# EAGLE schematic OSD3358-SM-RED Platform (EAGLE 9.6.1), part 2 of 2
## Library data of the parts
C1-C10 C12-C68 C70-C101 = OSD3358-SM-RED Platform:C: Capacitor SMD.
C11 C69 = OSD3358-SM-RED Platform:CPOL-US: POLARIZED CAPACITOR, American symbol
D1 D4-D7 D10 = OSD3358-SM-RED Platform:LTST-C191TBKT
D2 = OSD3358-SM-RED Platform:SMCJ15CA
D3 = OSD3358-SM-RED Platform:B520C-13-F: Schottky barrier diode
D8 D9 = OSD3358-SM-RED Platform:TPD4E05U06-Q1
D11 = OSD3358-SM-RED Platform:RB751V40-115
F1 = OSD3358-SM-RED Platform:FUSE
FB1 FB2 FB4 FB5 = OSD3358-SM-RED Platform:BLM21AG151SN1D: INDUCTOR
FB3 FB6 = OSD3358-SM-RED Platform:MPZ2012S601AT000: INDUCTOR
FUD1-FUD6 = OSD3358-SM-RED Platform:FIDUCIAL
J1 J2 J7-J9 J11 J12 J15 = OSD3358-SM-RED Platform:826646-2: 2-pin 100 mil header
J3 = OSD3358-SM-RED Platform:826646-6: 6-pin 100 mil header; MPN: P125-1106A1BS116A1
J4 = OSD3358-SM-RED Platform:FTR-110-51-L-D-06
J5 J6 = OSD3358-SM-RED Platform:TH-2X23: 320030002
J10 = OSD3358-SM-RED Platform:TH-2X5: 320030002
J14 = OSD3358-SM-RED Platform:PJ-102BH: 2.5 mm Center Pin, 5.0 A, Right Angle, Through Hole, Tapered Pins, Dc Power Jack Connector
L1 = OSD3358-SM-RED Platform:CVH252009-4R7M
MGT1-MGT4 = OSD3358-SM-RED Platform:MOUNTING_HOLE: Chassis Mounting Hole w/GND connection ability
Q1 = OSD3358-SM-RED Platform:MMBT2907: PNP Transistror
Q2 = OSD3358-SM-RED Platform:MMBT3904LP-7B
R1-R168 = OSD3358-SM-RED Platform:R-US_: RESISTOR, American symbol
S1-S3 = OSD3358-SM-RED Platform:KMR231GLFS
TP1-TP4 TP9-TP17 TP21-TP24 TP27-TP30 = OSD3358-SM-RED Platform:TP: Test pad
TP5-TP8 TP18-TP20 TP25 TP26 = OSD3358-SM-RED Platform:TESTPAD/W_HOLE_1X1: Test point (Through hole)
U1 = OSD3358-SM-RED Platform:OSD3358-512M-BSM: Octavo Systems LLC OSD335x Family SiP: 21mm x 21mm, 1.27mm pitch 256 pin BGA contains AM3358, 512MB DDR3, TPS65217, TL5209, EEPROM and passives. Commerical Temperature: 0C to 85C.
U2 = OSD3358-SM-RED Platform:TPD4S012DRYR; DATASHEETURL: http://www.ti.com/lit/gpn/TPD4S012; FAMILY_NAME: ESD Solution; GENERIC_PART_NUMBER: TPD4S012; INDUSTRY_STD_PKG_TYPE: SON; MANUFACTURER: Texas Instruments; MANUFACTURER_PART_NUMBER: tpd4s012_dry_6; PACKAGE_DESIGNATOR: DRY; PIN_COUNT: 6; VENDOR: Texas Instruments
U3 = OSD3358-SM-RED Platform:SN74LVC1G07DCKRG4
U4 = OSD3358-SM-RED Platform:BU4240FVE-TR
U5 = OSD3358-SM-RED Platform:TLVH431NAMQDBZRVL
U6 = OSD3358-SM-RED Platform:SN74LVC2G241DCUR
U7 = OSD3358-SM-RED Platform:THGBMNG5D1LBAIT
U8 = OSD3358-SM-RED Platform:USB2534-1080AEN
U9 = OSD3358-SM-RED Platform:AR8035-AL1A: Ethernet PHY (10/100/1000)
U10 = OSD3358-SM-RED Platform:TDA19988BHN/C1,551
U11-U14 = OSD3358-SM-RED Platform:TPD4S012DRYR
U15 = OSD3358-SM-RED Platform:TPS2051BDGN
U16 = OSD3358-SM-RED Platform:AT97SC3205T-G3M4400B: Trusted Platform Module
U17 = OSD3358-SM-RED Platform:TMP468AIYFFR
U18-U20 U24 = OSD3358-SM-RED Platform:SN74LVC2G53YZPR
U21 = OSD3358-SM-RED Platform:S25FL127S: Cypress Semiconductor S25FL127S http://www.cypress.com/file/177961/download https://www.digikey.com/product-detail/en/cypress-semiconductor-corp/S25FL127SABNFI101/1274-1046-ND/4142072
U22 = OSD3358-SM-RED Platform:LPS22HBTR: Pressure Sensor 3.77PSI ~ 18.27PSI (26kPa ~ 126kPa) Absolute 24 b 10-WFLGA Exposed Pad Check prices; AVAILABILITY: Good; DESCRIPTION: Pressure Sensor 3.77PSI ~ 18.27PSI (26kPa ~ 126kPa) Absolute 24 b 10-WFLGA Exposed Pad; MF: STMicroelectronics; MP: LPS22HBTR; PACKAGE: WFLGA-10 STMicroelectronics; PRICE: None; PURCHASE-URL: https://pricing.snapeda.com/search/part/LPS22HBTR/?ref=eda
U23 = OSD3358-SM-RED Platform:ICM-20948; MPN: ICM-20948
U25 = OSD3358-SM-RED Platform:PCA9306DQER: Check prices; AVAILABILITY: Good; DESCRIPTION: 2-bit bidirectional I2C bus and SMBus voltage-level shifter 8-X2SON -40 to 85; MF: Texas Instruments; MP: PCA9306DQER; PACKAGE: X2SON-8 Texas Instruments; PRICE: None; PURCHASE-URL: https://pricing.snapeda.com/search/part/PCA9306DQER/?ref=eda
U26 = OSD3358-SM-RED Platform:TPS22958DGKR
X1 = OSD3358-SM-RED Platform:10118192-0001LF: Amphenol FCI Micro USB Type B Complete Surface Mount (SMT) no guide holes
X3 = OSD3358-SM-RED Platform:DM3BT-DSF-PEJS: HIROSE - microSD Card socket - Reverse on-Board - Push / Push
X4 = OSD3358-SM-RED Platform:1002-004-01010: Dual USB connector (Horizontal)
X5 = OSD3358-SM-RED Platform:RJMG2310228A0ER
X6 = OSD3358-SM-RED Platform:10118241-001RLF: Micro-HDMI connector
Y1 = OSD3358-SM-RED Platform:ABS07-32.768KHZ-T: 32kHz crystal
Y2 Y4 = OSD3358-SM-RED Platform:7A-24.000MAAJ-T
Y3 = OSD3358-SM-RED Platform:ASDMB-12.000MHZ-LC-T: 12 MHz ocillator
Y5 = OSD3358-SM-RED Platform:ASDMB-24.576MHZ-LC-T
Y6 = OSD3358-SM-RED Platform:7A-25.000MAAE-T: 25MHz crystal

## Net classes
0 default: width 0.127 mm, drill 0.254 mm
1 ground: width 0.152 mm, drill 0.254 mm, clearance 0.152 mm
